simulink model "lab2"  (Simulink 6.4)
settings: Solver=ode45  StartTime=0.0  StopTime=10.0  RelTol=1e-3
undefined symbols (not defined in the file or in its folder): sfunyst

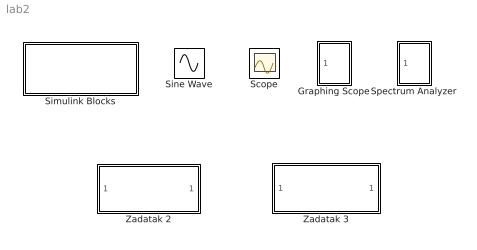
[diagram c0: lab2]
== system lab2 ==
  Graphing Scope : Subsystem  mask(Storage scope.){}
      mask help: Storage scope using MATLAB graph window. Enter plotting ranges and line type.
      mask init:
      | npts = @4; color = @5; ax = [0, @1, @2, @3]; dt=-1;
  Scope : Scope
  Simulink Blocks : Subsystem
  Sine Wave : Sin  SampleTime=0
  Spectrum Analyzer : Subsystem  mask(Spectrum analyzer.){}
      mask init:
      | N=@1; T_s=@2;plot_period=@3;
  Zadatak 2 : ModelReference  ModelName=lab2Synth  ModelReferenceVersion=1.2  CopyOfModelName=lab2Synth
  Zadatak 3 : ModelReference  ModelName=lab2Mod  ModelReferenceVersion=1.2  CopyOfModelName=lab2Mod

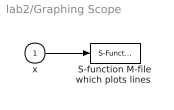
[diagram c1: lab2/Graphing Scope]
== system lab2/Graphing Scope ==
  x : Inport
  "S-function M-file which plots lines " : S-Function  LoadFcn=sfunyst([],[],[],'LoadBlock')  FunctionName=sfunyst  Parameters=ax, color, npts, dt
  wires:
  x/1 -> "S-function M-file which plots lines "/1

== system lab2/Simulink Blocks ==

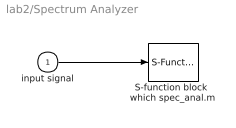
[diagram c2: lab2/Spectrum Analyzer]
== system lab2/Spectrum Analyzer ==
  input signal : Inport
  S-function block  which spec_anal.m : S-Function  FunctionName=SpecAnal  Parameters=N,T_s,plot_period
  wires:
  input signal/1 -> S-function block  which spec_anal.m/1
